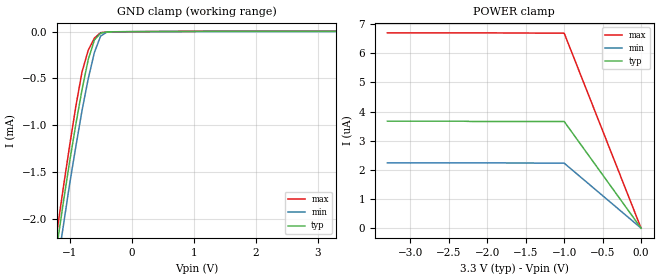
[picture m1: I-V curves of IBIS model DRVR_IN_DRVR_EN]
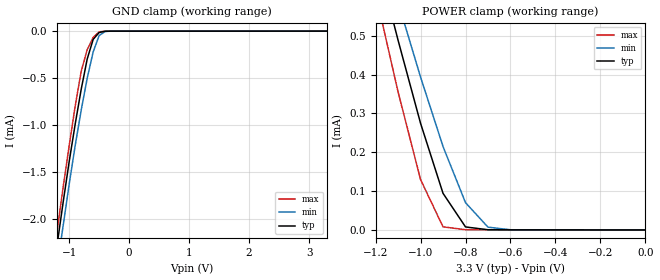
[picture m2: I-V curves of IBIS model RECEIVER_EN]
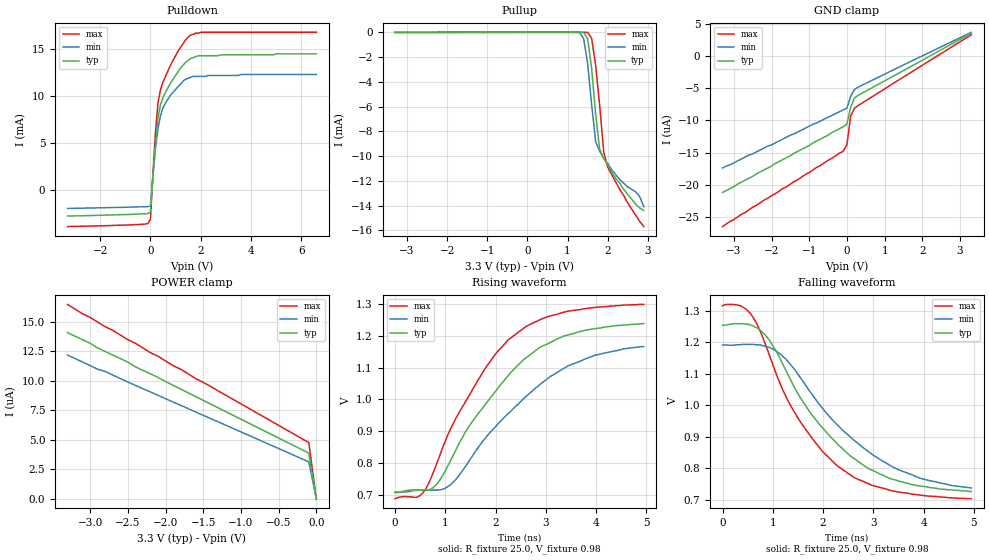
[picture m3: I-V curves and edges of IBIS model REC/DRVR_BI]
|   Texas Instruments Incorporated
|   Data Transmissions Products
|   IBIS Model for SN65MLVD200A
|   8D SOIC Package
[IBIS Ver]   3.2
[Comment char]   |_char
[File name]   mlvd200a.ibs
[File Rev]   1.0
[Date]   07Dec03
[Source]   File originated at Texas Instruments Incorporated.
   Data Transmission Products Group. All data based on
   Simulation Measurements.
[Notes]
[Disclaimer]
(C) Copyright Texas Instruments Incorporated 2003
   All rights reserved
  Texas Instruments Incorporated hereby grants the user of this IBIS
model a non-exclusive, nontransferable license to use this IBIS model
under the following terms.  Before using this IBIS model, the user
should read this license.  If the user does not accept these terms,
the IBIS model should be returned to Texas Instruments within 30 days.
  The user is granted this license only to use the IBIS model and
is not granted rights to sell, load, rent, lease or license the IBIS
model in whole or in part, or in modified form to anyone other than
user.  User may modify the IBIS model to suit its specific applications
but rights to derivative works and such modifications shall belong to
Texas Instruments.
  This IBIS model is provided on an "AS IS" basis and Texas Instruments
makes absolutely no warranty with respect to the information contained
herein.  TEXAS INSTRUMENTS DISCLAIMS AND CUSTOMER WAIVES ALL WARRANTIES,
EXPRESS OR IMPLIED, INCLUDING WARRANTIES OF MERCHANTABILITY OR FITNESS
FOR A PARTICULAR PURPOSE. The entire risk as to quality and performance
is with the Customer. ACCORDINGLY, IN NO EVENT SHALL THE COMPANY BE LIABLE
FOR ANY DAMAGES, WHETHER IN CONTRACT OR TORT,INCLUDING ANY LOST PROFITS
OR OTHER INCIDENTAL, CONSEQUENTIAL, EXEMPLARY, OR PUNITIVE DAMAGES ARISING
OUT OF THE USE OR APPLICATION OF THE IBIS model provided in this package.
Further, Texas Instruments reserves the right to discontinue or make changes
without notice to any product herein to improve reliability, function, or
design. Texas Instruments does not convey any license under patent rights
or any other intellectual property rights, including those of third parties.
Contact Texas Instruments at ATTN:DATA TRANSMISSIONS
[Copyright]   Copyright 2003, Texas Instruments, All Rights Reserved
[Component]   SN65MLVD200AD
[Manufacturer]  Texas Instruments Incorporated
[Package]
|   typ   min   max
R_pkg   0.036   0.033   0.039
L_pkg   3.340nH   2.445nH   4.233nH
C_pkg   0.470pF   0.308pF   0.631pF
[Pin]   signal_name   model_name   R_pin   L_pin   C_pin
1   R   RECEIVER_OUT   0.034   4.233n   0.630p
2   RE   RECEIVER_EN   0.038   2.445n   0.309p
3   DE   DRVR_IN_DRVR_EN   0.039   2.448n   0.309p
4   D   DRVR_IN_DRVR_EN   0.033   4.231n   0.631p
5   GND   GND   0.033   4.230n   0.630p
6   A   REC/DRVR_BI   0.039   2.450n   0.308p
7   B   REC/DRVR_BI   0.039   2.448n   0.309p
8   VCC   POWER   0.033   4.231n   0.630p
[Diff_pin]   inv_pin   vdiff   tdelay_typ   tdelay_min   tdelay_max
| The 'A' pin is Diff_pin and the 'B' pin is the inv_pin
   6   7   0.050   0   0   0
| Models and submodels in the file (4): DRVR_IN_DRVR_EN (Input), RECEIVER_EN (Input), REC/DRVR_BI (I/O), RECEIVER_OUT (3-state)
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|   Driver/Driver Enable Model
[Model]   DRVR_IN_DRVR_EN
Model_type   Input
|Signals   D,DE
Vinh = 2.0
Vinl = 0.8
|   typ   min   max
C_comp   3.78pF   3.55pF   3.91pF
|   typ   min   max
[Temperature Range]   25.0   85   -40
[Voltage range]   3.3V   3.0V   3.6V
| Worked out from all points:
|   GND clamp passes 1 mA (typ) near -0.90 V on its own axis
[GND_clamp]
|   Voltage   I(typ)   I(min)   I(max)
-3.3V     -14.3mA    -13.8mA    -14.9mA
-1.2V     -2.27mA    -2.51mA    -2.12mA
-1.1V     -1.82mA    -2.07mA    -1.66mA
-1V       -1.39mA    -1.63mA    -1.22mA
-900mV    -992uA     -1.23mA    -800uA
-800mV    -621uA     -844uA     -431uA
-700mV    -299uA     -504uA     -199uA
-600mV    -88.7uA    -222uA     -68.8uA
-500mV    -15.9uA    -47.1uA    -10.1uA
-400mV    -2.37uA    -4.7uA     -2.62uA
-300mV    -1.1uA     -932nA     -1.79uA
3.3V      3.66uA     2.23uA     6.68uA
[Power_clamp]
| Note that the[POWER_clamp]voltage table is referenced to Vcc
| and is calculated using Vtable=Vcc - Vmeasured.
|   Voltage   I(typ)   I(min)   I(max)
-3.3V     3.67uA     2.24uA     6.7uA
-2V       3.66uA     2.24uA     6.7uA
-1V       3.66uA     2.23uA     6.69uA
0V        0A         0A         0A
|   Receiver Enable Model
[Model]   RECEIVER_EN
Model_type   Input
|Signals   RE
Vinh = 2.0
Vinl = 0.8
|   typ   min   max
C_comp   3.76pF   3.56pF   3.93pF
|   typ   min   max
[Temperature Range]   25.0   85   -40
[Voltage range]   3.3V   3.0V   3.6V
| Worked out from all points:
|   GND clamp passes 1 mA (typ) near -0.90 V on its own axis
|   POWER clamp passes 1 mA (typ) near -1.32 V on its own axis
[GND_clamp]
|   Voltage   I(typ)   I(min)   I(max)
-3.3V     -14.3mA    -13.8mA    -14.9mA
-1.2V     -2.27mA    -2.51mA    -2.12mA
-1.1V     -1.82mA    -2.07mA    -1.66mA
-1V       -1.39mA    -1.63mA    -1.22mA
-900mV    -991uA     -1.22mA    -799uA
-800mV    -621uA     -843uA     -429uA
-700mV    -298uA     -503uA     -198uA
-600mV    -87.7uA    -221uA     -67uA
-500mV    -14.9uA    -46.5uA    -7.98uA
-400mV    -1.52uA    -4.17uA    -1.02uA
-300mV    -611nA     -639nA     -827nA
3.3V      64.2pA     131nA      -188nA
[Power_clamp]
| Note that the[POWER_clamp]voltage table is referenced to Vcc
| and is calculated using Vtable=Vcc - Vmeasured.
|   Voltage   I(typ)   I(min)   I(max)
-3.3V     5.83mA     5.29mA     6.46mA
-1.2V     714uA      787uA      610uA
-1.1V     489uA      587uA      356uA
-1V       275uA      394uA      130uA
-900mV    94.4uA     215uA      8.06uA
-800mV    7.83uA     70.3uA     643nA
-700mV    564nA      7.24uA     510nA
-600mV    340nA      574nA      435nA
0V        64.2pA     165pA      63.7pA
|   Driver Output/Receiver Input Model
[Model]   REC/DRVR_BI
Model_type   I/O
| Signals   A,B
Vinl = 1.15V
Vinh = 1.35V
Vmeas = 1.0   |Reference voltage for timing measurements
Cref = 2pF   |Timing specification test load capacitance value
Rref = 25   |Note: 25 Ohm load; single ended configuration
| variable   typ   min   max
C_comp   3.54pF   3.29pF   3.96pF
|   typ   min   max
[Temperature Range]   25.0   85   -40
[Voltage range]   3.3V   3.0V   3.6V
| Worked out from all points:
|   slope of the pulldown table from 0 to 0.495 V, typ, clamps not added: 40.6 ohm
|   rising waveform, R_fixture 25.0, V_fixture 0.98: 20-80 % time 1.5ns typ, 1.67ns min, 1.33ns max; typ from 0.706 V to 1.24 V
|   falling waveform, R_fixture 25.0, V_fixture 0.98: 20-80 % time 1.46ns typ, 1.64ns min, 1.31ns max; typ from 1.25 V to 0.726 V
[Pulldown]
|   Voltage   I(typ)   I(min)   I(max)
-3.3V     -2.8mA     -1.99mA    -3.92mA
-100mV    -2.53mA    -1.79mA    -3.59mA
0V        -2.37mA    -1.73mA    -3.15mA
100mV     1.48mA     1.47mA     1.75mA
200mV     5.06mA     4.39mA     6.18mA
300mV     7.66mA     6.52mA     9.23mA
400mV     9.09mA     7.91mA     10.7mA
500mV     9.85mA     8.75mA     11.5mA
800mV     11.4mA     10.1mA     13.3mA
1.5V      13.8mA     11.9mA     16.3mA
2V        14.3mA     12.1mA     16.8mA
6.6V      14.5mA     12.3mA     16.8mA
[Pullup]
|   Voltage   I(typ)   I(min)   I(max)
| Note that the[Pullup]voltage table is referenced to Vcc
| and is calculated using Vtable=Vcc - Vmeasured.
-3.3V     800nA      10nA       -16.5uA
1.3V      29nA       -14uA      2.6nA
1.4V      -4.43uA    -509uA     1.3nA
1.5V      -513uA     -2.52mA    -882nA
1.6V      -2.93mA    -5.83mA    -485uA
1.7V      -6.62mA    -8.84mA    -2.69mA
1.8V      -9.45mA    -9.61mA    -5.9mA
1.9V      -10.2mA    -10.2mA    -9.66mA
2V        -10.7mA    -10.6mA    -10.9mA
2.3V      -12.2mA    -11.9mA    -12.7mA
2.7V      -13.9mA    -12.9mA    -14.8mA
2.9V      -14.4mA    -14.1mA    -15.7mA
[GND_clamp]
|   Voltage   I(typ)   I(min)   I(max)
| Outputs in High Impedance (off)
-3.3V     -21.2uA    -17.4uA    -26.5uA
-100mV    -11uA      -8.38uA    -14.8uA
0V        -10.6uA    -8.1uA     -13.8uA
100mV     -7.96uA    -6.25uA    -9.33uA
200mV     -6.52uA    -5.19uA    -8.12uA
300mV     -6.1uA     -4.82uA    -7.68uA
3.3V      3.55uA     3.69uA     3.31uA
[Power_clamp]
| Note that the[POWER_clamp]voltage table is referenced to Vcc
| and is calculated using Vtable=Vcc - Vmeasured.
|   Voltage   I(typ)   I(min)   I(max)
-3.3V     14.1uA     12.2uA     16.5uA
-3.1V     13.5uA     11.6uA     15.7uA
-3V       13.2uA     11.3uA     15.4uA
-2.9V     12.8uA     11uA       15uA
-2.8V     12.5uA     10.8uA     14.6uA
-2.7V     12.2uA     10.5uA     14.3uA
-2.5V     11.6uA     9.91uA     13.5uA
-2.4V     11.2uA     9.62uA     13.2uA
-2.2V     10.6uA     9.06uA     12.4uA
-1.6V     8.67uA     7.36uA     10.2uA
-100mV    3.87uA     3.13uA     4.77uA
0V        0A         0A         0A
[Ramp]
|   typ   min   max
dV/dt_r   0.326/1.568ns   0.286/1.817ns   0.375/1.381ns
dV/dt_f   0.325/1.550ns   0.285/1.798ns   0.375/1.371ns
R_load = 25ohm  | Note: The measurement is single-ended with 25ohm
|   to ground.
[Rising Waveform]
R_fixture = 25.0
V_fixture = 0.98
V_fixture_min = 0.95
V_fixture_max = 1.00
C_fixture = 0p
L_fixture = 0n
|   V(typ)   V(min)   V(max)
0s        706mV      708mV      687mV
500ps     714mV      714mV      697mV
850ps     736mV      714mV      806mV
1.3ns     868mV      766mV      965mV
1.8ns     985mV      878mV      1.099V
2.25ns    1.074V     955mV      1.187V
2.85ns    1.16V      1.042V     1.248V
3.35ns    1.199V     1.097V     1.274V
4ns       1.223V     1.14V      1.29V
4.95ns    1.239V     1.166V     1.299V
[Falling Waveform]
R_fixture = 25.0
V_fixture = 0.98
V_fixture_min = 0.95
V_fixture_max = 1.00
C_fixture = 0p
L_fixture = 0n
|   V(typ)   V(min)   V(max)
0s        1.254V     1.191V     1.316V
500ps     1.257V     1.193V     1.3V
650ps     1.248V     1.192V     1.268V
850ps     1.223V     1.187V     1.195V
1.2ns     1.13V      1.155V     1.048V
1.5ns     1.037V     1.098V     959mV
2.3ns     874mV      935mV      805mV
2.9ns     799mV      853mV      751mV
3.5ns     759mV      795mV      724mV
4.95ns    726mV      737mV      703mV
